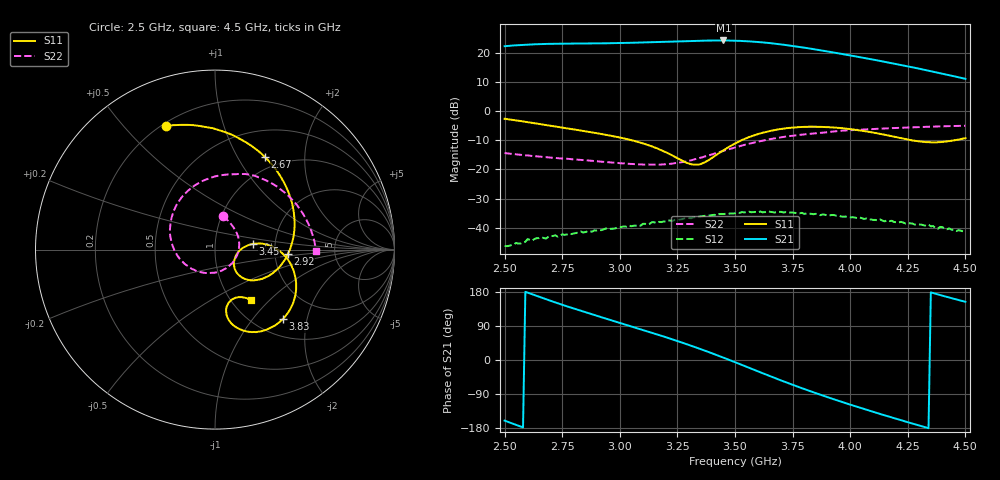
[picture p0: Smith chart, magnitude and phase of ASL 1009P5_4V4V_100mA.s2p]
!ASL 1009P5 : Low Noise Amplifier S-parameter data 2.5-4.5 GHz
!Bias conditions Vd1=4V, Vd2=4V, Total current=100 mA
!Date: Tuesday, January 09, 2007 14:21:38
!S2P File: Measurements: S11, S21, S12, S22:
# Hz S  dB  R 50
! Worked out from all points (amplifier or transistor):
!   201 points, 2.5 GHz to 4.5 GHz, reference 50 ohm
!   highest |S21| = 24.3 dB at 3.45 GHz (marker M1)
!   |S21| within 3 dB of that: start of sweep to 3.843 GHz
!   unconditionally stable (mu >= 1): start of sweep to end of sweep
!   at 2.83 GHz: K = 3.17, MAG = 24.3 dB, |S12| = -41.2 dB
!   at 3.5 GHz: K = 1.67, MAG = 24.8 dB, |S12| = -35.0 dB
!   at 4.5 GHz: K = 9.77, MAG = 13.4 dB, |S12| = -41.4 dB
!   S11 on the Smith chart (normalised r, x): 2.5 GHz: 0.22, +0.66; 2.67 GHz: 0.83, +1.31; 2.92 GHz: 2.36, -0.15; 3.45 GHz: 1.53, +0.10; 3.83 GHz: 1.32, -1.44; 4.5 GHz: 1.22, -0.78
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2.5e9  -2.61 111.4  22.28 -160.0  -46.26 119.6  -14.36 76.5
2.59e9  -3.64 85.2  22.80 179.9  -44.83 101.0  -15.16 64.6
2.67e9  -4.64 61.8  23.05 162.5  -43.54 85.4  -15.72 53.5
2.74e9  -5.52 41.8  23.16 147.8  -42.82 74.4  -16.20 42.7
2.84e9  -6.76 15.2  23.22 128.0  -41.61 54.2  -16.74 24.9
2.92e9  -7.83 -3.7  23.28 112.9  -40.85 44.7  -17.32 8.5
3.04e9  -9.77 -27.9  23.45 90.6  -39.22 22.7  -18.07 -21.1
3.17e9  -13.05 -45.4  23.74 66.0  -37.97 -2.2  -18.36 -62.7
3.31e9  -18.21 -29.2  24.10 37.6  -36.74 -27.0  -16.84 -116.7
3.38e9  -17.06 -0.9  24.21 22.3  -35.81 -42.5  -15.30 -143.6
3.45e9  -13.42 8.6  24.26 6.2  -35.29 -59.4  -13.62 -168.7
3.5e9  -11.09 6.2  24.18 -5.8  -35.04 -71.9  -12.45 174.2
3.58e9  -8.37 -3.9  23.84 -25.1  -34.64 -89.8  -10.82 149.4
3.67e9  -6.50 -18.9  23.20 -46.9  -34.74 -111.8  -9.35 124.6
3.74e9  -5.71 -31.0  22.49 -63.1  -34.79 -126.8  -8.52 107.5
3.83e9  -5.33 -45.7  21.42 -83.0  -35.21 -145.6  -7.73 88.2
3.84e9  -5.34 -47.3  21.30 -85.1  -35.37 -147.6  -7.64 86.1
3.92e9  -5.56 -58.6  20.24 -101.8  -35.61 -164.4  -7.04 71.3
4e9  -6.14 -68.1  19.13 -117.7  -36.45 179.4  -6.53 58.3
4.17e9  -8.45 -79.7  16.62 -149.7  -37.72 150.7  -5.87 34.6
4.33e9  -10.63 -71.8  14.08 -178.3  -39.33 123.8  -5.37 16.1
4.5e9  -9.25 -54.8  11.09 153.6  -41.41 97.7  -4.99 -0.9
